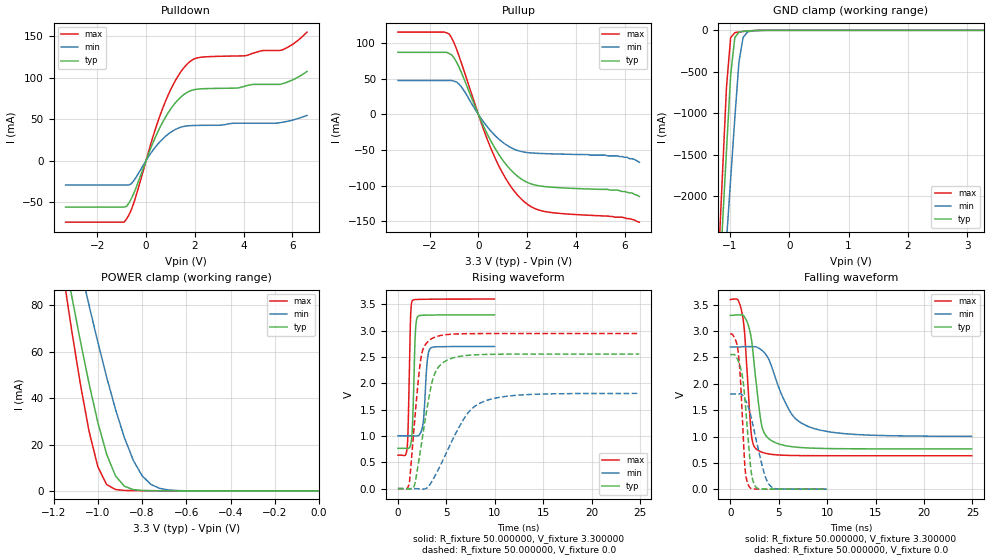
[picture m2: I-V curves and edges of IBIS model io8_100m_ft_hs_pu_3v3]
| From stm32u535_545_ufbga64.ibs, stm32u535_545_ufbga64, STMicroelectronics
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|   Model io8_100m_ft_hs_pu_3v3
[Model]  io8_100m_ft_hs_pu_3v3
Model_type I/O
Polarity   Non-Inverting
Enable   Active-Low
Vinl =   0.990000V
Vinh =   2.310000V
Vmeas =  1.650000V
Cref =   50.000000pF
Rref =   100.000000M
Vref =   0.0V
C_comp   3.313100pF   3.281800pF   3.354500pF
[Temperature Range]   25.000000   0.140000k   -40.000000
[Pullup Reference]   3.300000V   2.700000V   3.600000V
[Pulldown Reference]   0.0V   0.0V   0.0V
[POWER Clamp Reference]   3.300000V   2.700000V   3.600000V
[GND Clamp Reference]   0.0V   0.0V   0.0V
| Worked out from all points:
|   slope of the pulldown table from 0 to 0.495 V, typ, clamps not added: 14 ohm
|   slope of the pullup table from 0 to 0.495 V, typ, clamps not added: 13.7 ohm
|   GND clamp passes 1 mA (typ) near -0.51 V on its own axis
|   POWER clamp passes 1 mA (typ) near -0.85 V on its own axis
|   rising waveform, R_fixture 50.000000, V_fixture 3.300000: 20-80 % time 244ps typ, 341ps min, 207ps max; typ from 0.765 V to 3.3 V
|   rising waveform, R_fixture 50.000000, V_fixture 0.0: 20-80 % time 1.41ns typ, 3.1ns min, 871ps max; typ from 0.001 V to 2.55 V
|   falling waveform, R_fixture 50.000000, V_fixture 3.300000: 20-80 % time 960ps typ, 2.52ns min, 626ps max; typ from 3.3 V to 0.765 V
|   falling waveform, R_fixture 50.000000, V_fixture 0.0: 20-80 % time 726ps typ, 1.36ns min, 504ps max; typ from 2.55 V to 0.001 V
[Pulldown]
|Voltage   I(typ)   I(min)   I(max)
-3.3V     -56.06mA   -29.42mA   -74.35mA
-900mV    -56.06mA   -29.42mA   -74.35mA
-700mV    -51.09mA   -29.42mA   -65.48mA
-500mV    -39.32mA   -24.2mA    -50.88mA
300mV     22.62mA    13.13mA    30.42mA
800mV     52.54mA    29.36mA    71.75mA
1.3V      72.91mA    38.82mA    101.4mA
1.8V      84.02mA    42.13mA    119.4mA
2.3V      86.61mA    42.5mA     124.8mA
5.5V      91.97mA    45.76mA    132.8mA
6V        97.2mA     48.8mA     140mA
6.6V      107.6mA    54.5mA     155mA
[Pullup]
|Voltage   I(typ)   I(min)   I(max)
-3.3V     87.15mA    47.7mA     115.5mA
-1.2V     85.45mA    47.7mA     112.8mA
-1V       79.36mA    46.62mA    100.4mA
-700mV    59.07mA    38.77mA    72.39mA
200mV     -15.65mA   -9.933mA   -19.95mA
700mV     -48.51mA   -30.11mA   -62.22mA
1.3V      -76.68mA   -45.83mA   -99.4mA
1.9V      -93.37mA   -52.9mA    -122.9mA
2.3V      -98.71mA   -54.23mA   -131.6mA
2.8V      -101.3mA   -54.97mA   -136.5mA
5.7V      -106mA     -58mA      -144mA
6.6V      -115mA     -67mA      -151mA
[GND_clamp]
|Voltage   I(typ)   I(min)   I(max)
-3.3V     -9.848A    -9.957A    -9.458A
-1.2V     -3.312A    -4.013A    -2.863A
-1.13V    -2.381A    -3.274A    -1.769A
-1.06V    -1.452A    -2.535A    -684.7mA
-990mV    -542.9mA   -1.798A    -88.02mA
-920mV    -87.11mA   -1.064A    -28.44mA
-850mV    -22.1mA    -382.4mA   -19.61mA
-780mV    -11.97mA   -86.98mA   -13.71mA
-710mV    -7.619mA   -22.26mA   -8.745mA
-640mV    -4.493mA   -7.773mA   -4.817mA
-360mV    -31.22uA   -172.6uA   -8.607uA
3.28V     0A         15.66nA    -5.841nA
[POWER_clamp]
|Voltage   I(typ)   I(min)   I(max)
-3.28V    1.355A     1.167A     1.665A
-1.16V    105.8mA    131.6mA    95.87mA
-1.12V    85.08mA    114mA      70.45mA
-1.08V    65.19mA    96.88mA    46.75mA
-1.04V    46.48mA    80.2mA     25.96mA
-1V       29.64mA    64.18mA    10.49mA
-960mV    15.81mA    49.06mA    2.743mA
-920mV    6.481mA    35.16mA    612.9uA
-840mV    578.2uA    13.29mA    138.5uA
-760mV    94.37uA    2.807mA    98.56uA
-640mV    40.55uA    159.2uA    59.96uA
0V        0A         19.29nA    0A
[Ramp]
| variable   typ   min   max
dV/dt_r  1.53214/1.41038n   1.08399/3.10070n   1.76624/0.86949n
dV/dt_f  1.52096/0.95581n   1.01748/2.50771n   1.77908/0.62417n
R_load = 50.000000
[Rising Waveform]
R_fixture= 50.000000
V_fixture= 3.300000
V_fixture_min= 2.700000
V_fixture_max= 3.600000
|time   V(typ)   V(min)   V(max)
0s        765.1mV    1.003V     634.9mV
961ps     760.9mV    1.003V     795.6mV
1.301ns   828mV      1.003V     3.225V
1.481ns   1.123V     1.002V     3.567V
1.782ns   2.89V      1V         3.59V
2.042ns   3.266V     1.003V     3.593V
2.563ns   3.292V     1.199V     3.595V
3.043ns   3.295V     2.446V     3.596V
3.363ns   3.296V     2.666V     3.597V
9.97ns    3.3V       2.7V       3.599V
[Rising Waveform]
R_fixture= 50.000000
V_fixture= 0.0
V_fixture_min= 0.0
V_fixture_max= 0.0
|time   V(typ)   V(min)   V(max)
0s        833uV      853.6uV    875.1uV
1.151ns   -7.905mV   865.6uV    88.03mV
1.702ns   61.56mV    847.3uV    1.231V
2.402ns   816.6mV    -8.019mV   2.507V
3.403ns   1.924V     106.7mV    2.838V
3.904ns   2.227V     267.9mV    2.882V
4.855ns   2.417V     623.2mV    2.921V
7.007ns   2.527V     1.381V     2.942V
8.809ns   2.547V     1.65V      2.944V
24.92ns   2.554V     1.808V     2.945V
[Falling Waveform]
R_fixture= 50.000000
V_fixture= 3.300000
V_fixture_min= 2.700000
V_fixture_max= 3.600000
|time   V(typ)   V(min)   V(max)
0s        3.3V       2.7V       3.599V
1.251ns   3.307V     2.705V     3.308V
1.502ns   3.26V      2.706V     2.919V
2.202ns   2.823V     2.706V     1.005V
2.853ns   1.732V     2.686V     739mV
3.303ns   1.167V     2.63V      699.7mV
3.904ns   971.1mV    2.488V     671.4mV
6.106ns   814mV      1.492V     641.2mV
7.958ns   783.7mV    1.196V     636.8mV
24.92ns   765.1mV    1.003V     634.9mV
[Falling Waveform]
R_fixture= 50.000000
V_fixture= 0.0
V_fixture_min= 0.0
V_fixture_max= 0.0
|time   V(typ)   V(min)   V(max)
0s        2.554V     1.808V     2.945V
800.8ps   2.444V     1.808V     2.631V
1.041ns   2.316V     1.811V     2.114V
1.522ns   1.687V     1.707V     407.8mV
1.962ns   699.7mV    1.505V     47.01mV
2.222ns   258.1mV    1.317V     8.259mV
2.523ns   76.47mV    1.065V     3.646mV
3.504ns   3.144mV    304.1mV    2.034mV
4.144ns   2.274mV    61.71mV    1.749mV
9.97ns    833uV      853.6uV    875.1uV
